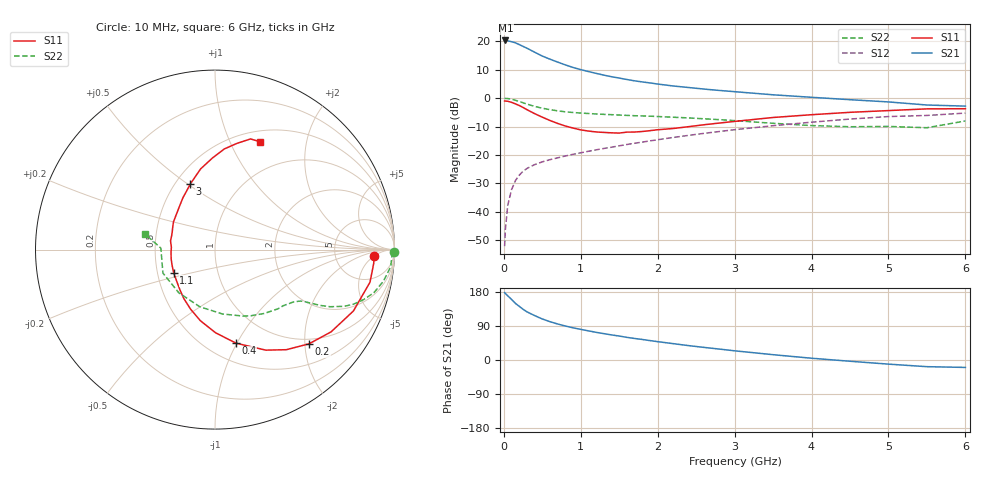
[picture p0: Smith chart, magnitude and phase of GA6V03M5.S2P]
! Infineon Technologies  Discrete & RF Semiconductors
! BF775
! Si NPN RF Bipolar Junction Transistor in SOT23
! VCE = 6 V  IC = 3.5 mA
! Common Emitter S-Parameters:  May  1996
# GHz  S  MA  R  50
!  f  S11  S21  S12  S22
! GHz  MAG  ANG  MAG  ANG  MAG  ANG  MAG  ANG
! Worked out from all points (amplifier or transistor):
!   36 points, 10 MHz to 6 GHz, reference 50 ohm
!   highest |S21| = 20.3 dB at 20 MHz (marker M1)
!   |S21| within 3 dB of that: start of sweep to 319.9 MHz
!   unconditionally stable (mu >= 1): 963.5 MHz to 3.262 GHz
!   at 250 MHz: K = 0.38, MSG = 21.9 dB, |S12| = -25.7 dB
!   at 1.4 GHz: K = 1.11, MAG = 10.3 dB, |S12| = -17.3 dB
!   at 6 GHz: K = 0.93, MSG = 1.2 dB, |S12| = -5.3 dB
!   S11 on the Smith chart (normalised r, x): 10 MHz: 15, -5; 200 MHz: 0.90, -2.09; 400 MHz: 0.68, -0.99; 1.1 GHz: 0.61, -0.17; 3 GHz: 0.59, +0.51; 6 GHz: 0.63, +1.31
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0.01  0.889 -2.4  10.19 177.9  0.0025 91.8  0.9963 -0.9
0.02  0.8874 -5.1  10.32 175.4  0.0049 90.2  0.9861 -2.2
0.05  0.8824 -11.9  10.18 169.6  0.0129 82.2  0.9837 -5.5
0.1  0.8437 -23.9  9.814 159.9  0.0246 76.9  0.955 -10.6
0.15  0.7928 -35.3  9.393 149.5  0.0354 70.4  0.9171 -15.2
0.2  0.742 -45.0  8.738 141.6  0.0442 66.4  0.8737 -18.6
0.25  0.685 -54.5  8.122 133.9  0.0519 62.6  0.8295 -21.5
0.3  0.6276 -63.2  7.548 127.2  0.058 60.1  0.7862 -23.7
0.4  0.534 -77.4  6.425 117.2  0.0678 55.9  0.716 -26.4
0.5  0.4629 -89.7  5.481 108.3  0.0759 54.3  0.6649 -27.9
0.6  0.4046 -101.6  4.838 101.1  0.083 53.2  0.6273 -28.8
0.7  0.359 -112.2  4.298 95.0  0.0893 53.3  0.5978 -29.6
0.9  0.2978 -130.9  3.459 84.9  0.1029 53.6  0.5589 -30.9
1.1  0.2639 -150.7  2.932 76.9  0.1164 54.1  0.5368 -32.7
1.3  0.2498 -167.8  2.538 69.6  0.1305 54.6  0.5188 -34.7
1.6  0.2527 168.7  2.124 59.7  0.1532 55.1  0.4974 -38.4
2.2  0.2924 137.1  1.636 43.2  0.2034 53.8  0.4618 -48.3
3  0.3897 110.8  1.299 24.2  0.2788 48.3  0.4024 -67.0
3.5  0.4568 100.1  1.144 14.0  0.3276 43.4  0.3613 -83.3
4.5  0.5633 84.7  0.939 -3.3  0.429 31.4  0.314 -129.9
5.5  0.6476 72.2  0.757 -17.6  0.4964 15.8  0.3018 178.4
6  0.6514 67.1  0.724 -19.6  0.546 11.5  0.3969 167.6
